FUNCTION_BLOCK FB700
TITLE =
//Call this FB as long as Done is FALSE. If Done is TRUE and Status is 0x0000, one
//packet has been sent without error. Then the source (anySource) can be
//recalculated. After that call this FB again.
//The following Status values are used:
//0x0000: packet has been sent without error
//0x8181: sending telegrams or waiting for response telegram
//0x8101: invalid length within anySource
//0x8182: invalid length within anySend
//0x8183: invalid length within anyRecv
//
//An instance DB has to be created before using this FB, clear the whole DB within
//OB100 (OB101, OB102) as initialization.
AUTHOR : ab_hk
FAMILY : AbvSpu
NAME : DL_SEND
VERSION : 0.1


VAR_INPUT
  anySource : ANY ;	//Pointer to source to be sent
  anySend : ANY ;	//Pointer to send buffer
  anyRecv : ANY ;	//Pointer to receive buffer
END_VAR
VAR_OUTPUT
  Done : BOOL ;	//TRUE if whole source (one packet) has been sent
  Error : BOOL ;	//TRUE if an error has been recognized
  Status : WORD ;	//Status Word indicating progress
END_VAR
VAR
  uchPrevSentPacketNo : BYTE ;
  uchPrevSentTeleNo : BYTE ;
  bOrderRunning : BOOL ;
END_VAR
VAR_TEMP
  uchRecvPacketNo : BYTE ;
  uchRecvTeleNo : BYTE ;
  wOldDB : WORD ;
  wNettoLen : WORD ;
  wOffset : WORD ;
  wTeleCount : WORD ;
  uchSendPacketNo : BYTE ;
  uchSendTeleNo : BYTE ;
  wActNettoLen : WORD ;
  wAct : WORD ;
  ptrSrc : DWORD ;
  ptrDst : DWORD ;
END_VAR
BEGIN
NETWORK
TITLE =

// total length to send: DIW  2
// send buffer length:   DIW 12
// recv buffer length:   DIW 22 (must be 2)

// check width of anySource:
      L     DIW    2;
      L     0;
      ==I   ;
      L     W#16#8101; // nothing to send
      SPB   err;

// check width of anySend:
      L     DIW   12;
      L     6;
      <=I   ;
      L     W#16#8102; // send buffer too short
      SPB   err;

// check width of anyRecv:
      L     DIW   22;
      L     2;
      <>I   ;
      L     W#16#8103; // recv buffer has other length than 2
      SPB   err;

// save DB register
      L     DBNO;
      T     #wOldDB;


// read incoming 2 bytes
      AUF   DB [DIW 24]; // DIW 24 may be 0
      LAR1  DID   26;
      L     B [AR1,P#0.0];
      T     #uchRecvPacketNo;
      L     B [AR1,P#1.0];
      T     #uchRecvTeleNo;

      L     #uchPrevSentPacketNo;
      SLW   8;
      L     #uchPrevSentTeleNo;
      +I    ;
      L     W [AR1,P#0.0]; // received bytes
      ==I   ;
      SPB   next; // received bytes are same as sent bytes, initially both 0 each

      L     W#16#8181; // pending
      T     #Status;
      CLR   ;
      =     #Done;
      =     #Error;
      SPA   end; // wait until echo received

next: NOP   0; // send next tele
      L     DIW   12;
      L     6;
      -I    ;
      T     #wNettoLen;


// calc wTeleCount:
      L     DIW    2; // total length to send
      +D    ; // + wNettoLen
      +     -1; // -1
      L     #wNettoLen;
      /I    ;
      T     #wTeleCount; // last tele filled with 0

// calc next tele number:
      T     #wTeleCount;
      L     #uchRecvTeleNo; // tele count already sent, initially 0
      INC   1; // next tele number
      <I    ; // last tele already sent?
      SPB   npck;
      T     #uchSendTeleNo;
      L     #uchRecvPacketNo;
      SPA   cpck;

npck: NOP   0; // next packet
      L     1;
      T     #uchSendTeleNo;

      L     #uchRecvPacketNo;
      +     1;
cpck: NOP   0; // check packet number
      T     #uchSendPacketNo;
      L     0;
      <>I   ;
      SPB   cntl;
      INC   1;
      T     #uchSendPacketNo;

cntl: NOP   0; // calc wActNettoLen:
      L     #uchSendTeleNo;
      L     #wTeleCount;
      <D    ;
      L     #wNettoLen;
      SPB   sntl;

      L     #wTeleCount;
      DEC   1;
      L     #wNettoLen;
      *I    ;
      L     DIW    2;
      TAK   ;
      -I    ;

sntl: NOP   0; // store wActNettoLen
      T     #wActNettoLen;

// check if next tele belongs to next packet
      UN    #bOrderRunning;
      SPB   cptr;
      L     #uchSendTeleNo;
      L     1;
      <>I   ;
      SPB   cptr;
      R     #bOrderRunning;
      R     #Error;
      SET   ;
      =     #Done;
      L     0;
      T     #Status;
      SPA   end;

cptr: NOP   0; // calc pointer to source
      SET   ;
      =     #bOrderRunning;
      LAR1  DID    6;
      L     #uchSendTeleNo;
      DEC   1;
      L     #wNettoLen;
      *D    ;
      SLW   3;
      +AR1  ; // source
      TAR1  ;
      T     #ptrSrc;

      LAR1  DID   16; // destination (send buffer)
      TAR1  ;
      T     #ptrDst;

      AUF   DB [DIW 14]; // open send buffer
// write header
      L     #ptrDst;
      LAR1  ;
      L     #uchSendPacketNo;
      T     B [AR1,P#0.0];

      L     #uchSendTeleNo;
      T     B [AR1,P#1.0];
      L     #wNettoLen;
      L     6;
      +I    ;
      T     W [AR1,P#2.0];
      +AR1  P#4.0;
      TAR1  ;
      T     #ptrDst;

// write data
      L     #wActNettoLen;
      T     #wAct;

lp1:  NOP   0; // loop for copying data
      AUF   DB [DIW 4];
      L     #ptrSrc;
      LAR1  ;
      L     B [AR1,P#0.0];
      AUF   DB [DIW 14];
      L     #ptrDst;
      LAR1  ;
      TAK   ;
      T     B [AR1,P#0.0];

      L     #ptrSrc;
      +     8; // P#1.0
      T     #ptrSrc;

      L     #ptrDst;
      +     8; // P#1.0
      T     #ptrDst;

      L     #wAct;
      DEC   1;
      T     #wAct;

      L     0;
      <>I   ;
      SPB   lp1;

// fill with zero and  write footer
      L     #wNettoLen;
      L     #wActNettoLen;
      -I    ;
      T     #wAct;
      SPZ   sptn;

      AUF   DB [DIW 14];
lp2:  NOP   0; // loop for filling with zero
      L     #ptrDst;
      LAR1  ;
      L     0;
      T     B [AR1,P#0.0];

      L     #ptrDst;
      +     8; // P#1.0
      T     #ptrDst;

      L     #wAct;
      DEC   1;
      T     #wAct;

      L     0;
      <>I   ;
      SPB   lp2;

sptn: NOP   0; // save packet and tele number
      AUF   DB [DIW 14]; // open receive buffer
// write footer and store previous numbers
      L     #ptrDst;
      LAR1  ;
      L     #uchSendPacketNo;
      T     B [AR1,P#0.0];
      T     #uchPrevSentPacketNo;

      L     #uchSendTeleNo;
      T     B [AR1,P#1.0];
      T     #uchPrevSentTeleNo;

      SPA   end;



err:  NOP   0; // any error
      T     #Status;
      SET   ;
      =     #Error;
      =     #Done;
      SPA   end;


end:  NOP   0;

      AUF   DB [#wOldDB]; // restore DB register
      BE    ;
END_FUNCTION_BLOCK

